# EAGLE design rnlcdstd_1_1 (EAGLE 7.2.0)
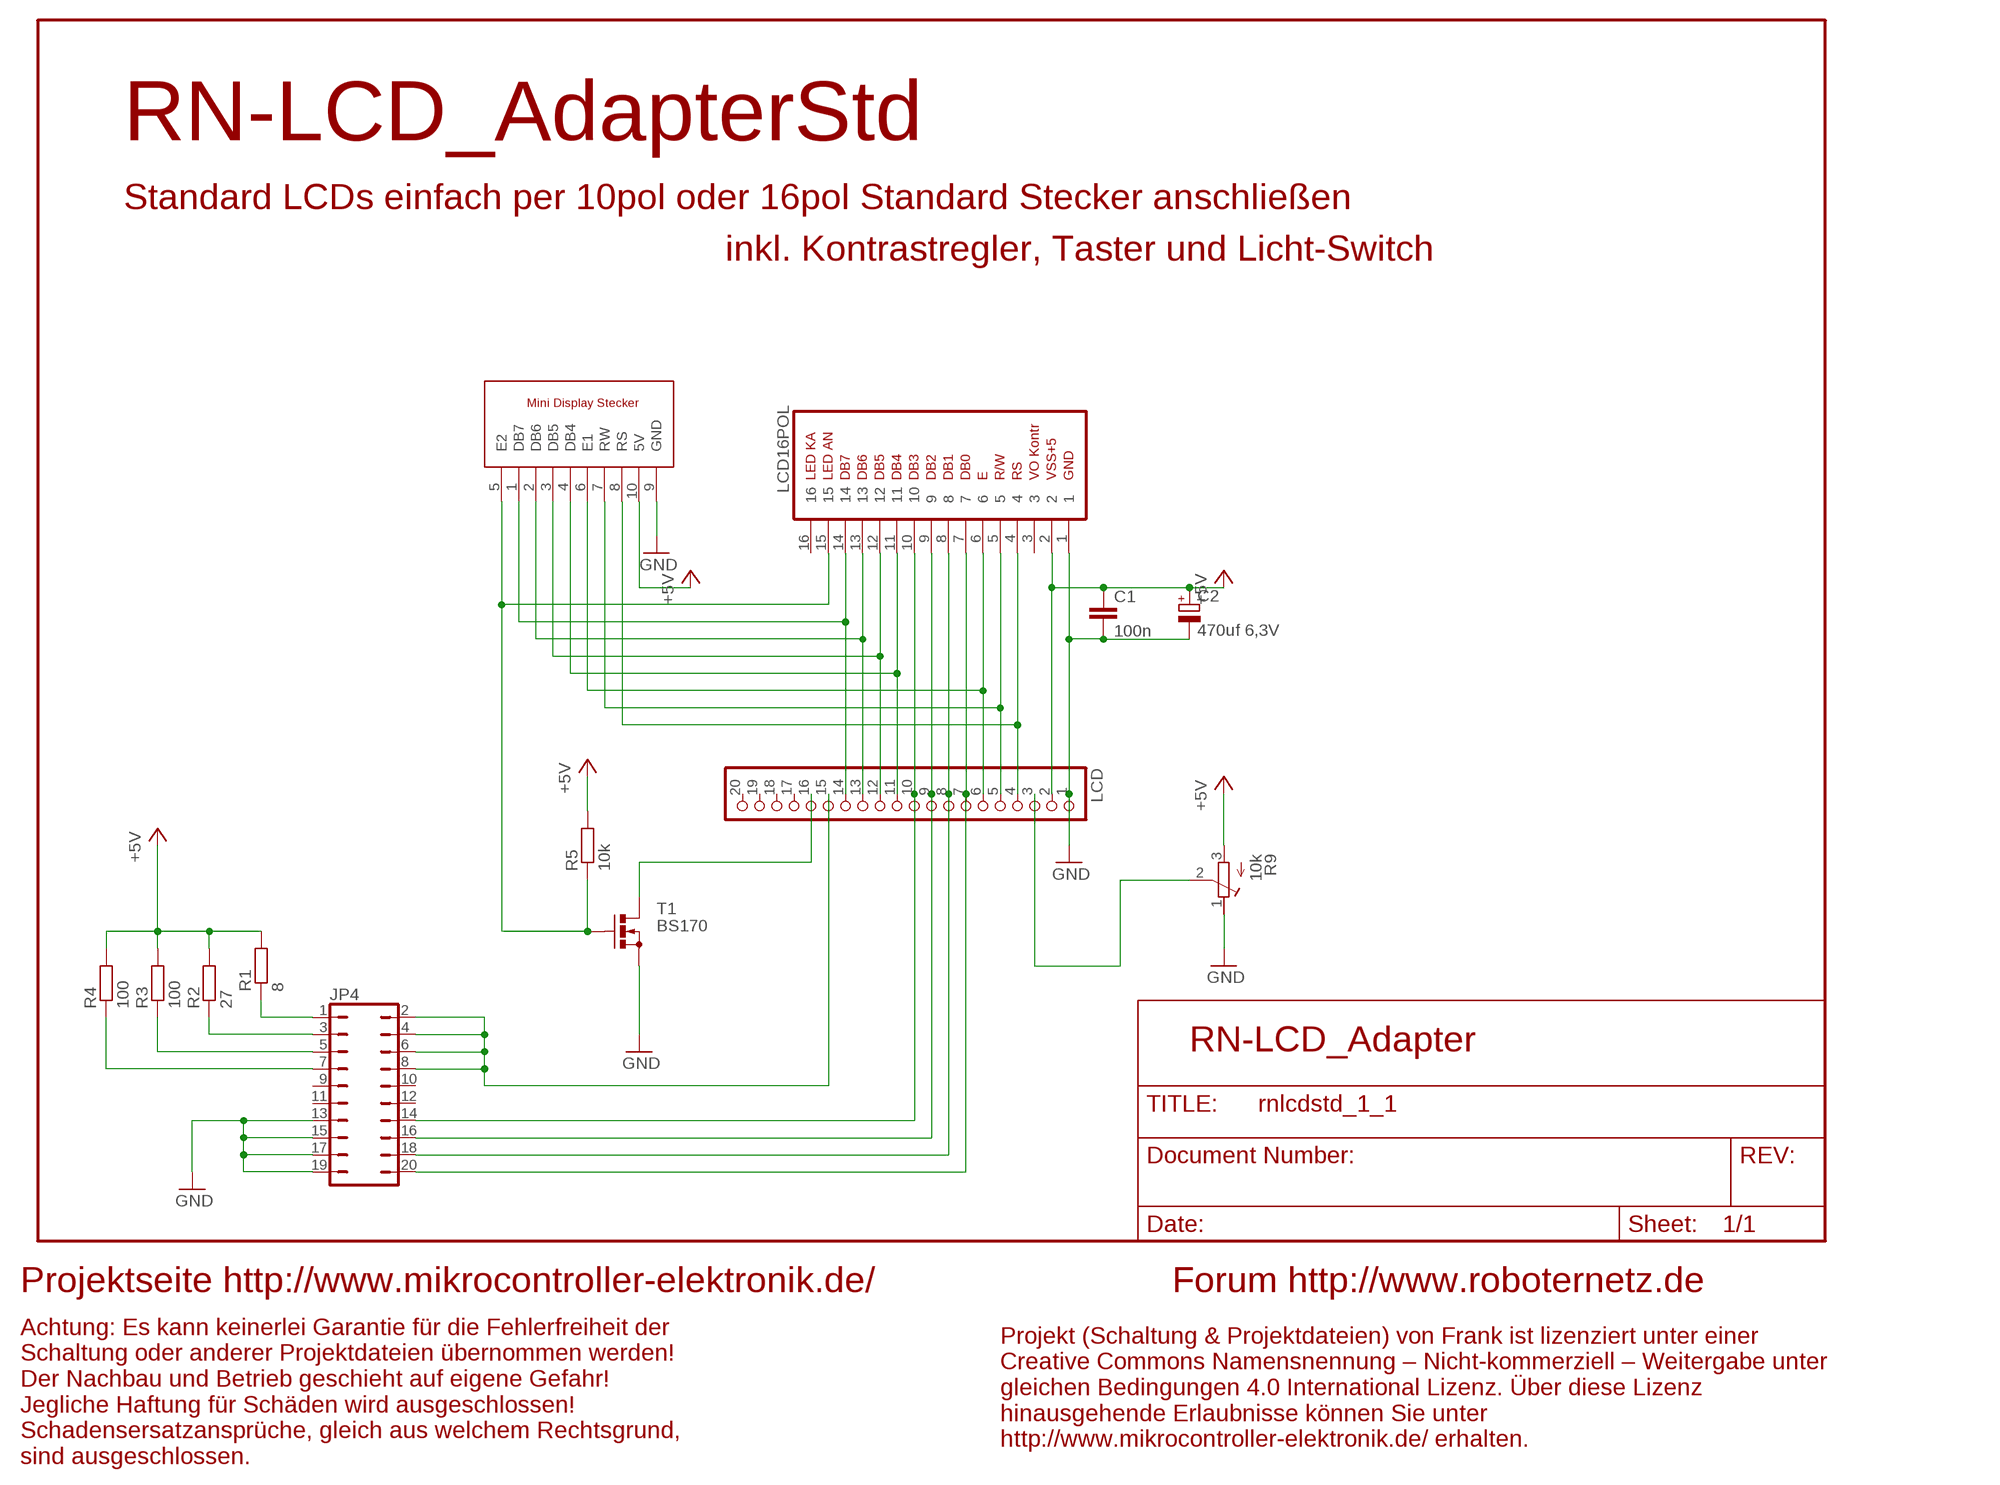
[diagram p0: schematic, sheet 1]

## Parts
C1  100n  C-EU050-024X044  [C050-024X044]
C2  470uf 6,3V  CPOL-EUE3.5-8  [E3,5-8]
JP4  JP10Q  [JP10Q]
LCD  PINHD-1X20  [1X20]
LCD4POL  DISPLAYSTECKER10PNEU  [ML10]
LCD16POL  DISPLAYSTECKER16P  [ML16]
R1  8  R-EU_0309/12  [0309/12]
R2  27  R-EU_0309/12  [0309/12]
R3  100  R-EU_0309/12  [0309/12]
R4  100  R-EU_0309/12  [0309/12]
R5  10k  R-EU_0207/10  [0207/10]
R9  10k  R-TRIMM43P  [RTRIM43P]
T1  BS170  [SOT54E]

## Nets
+5V [power]: C1.1 C2.+ LCD4POL.10(5V) LCD16POL.2 LCD.2 R1.2 R2.2 R3.2 R4.2 R5.2 R9.3(E)
GND [power]: C1.2 C2.- JP4.13 JP4.15 JP4.17 JP4.19 LCD4POL.9(GND) LCD16POL.1 LCD.1 R9.1(A) T1.S
N$1: LCD4POL.1(DB7) LCD16POL.14 LCD.14
N$2 [power]: LCD.16 T1.D
N$3: JP4.2 JP4.4 JP4.6 JP4.8 LCD.15
N$4: JP4.1 R1.1
N$5: LCD4POL.6(E1) LCD16POL.6 LCD.6
N$6: LCD4POL.8(RS) LCD16POL.4 LCD.4
N$7: LCD4POL.7(RW) LCD16POL.5 LCD.5
N$8: LCD.3 R9.2(S)
N$10: JP4.3 R2.1
N$11: JP4.5 R3.1
N$12: JP4.7 R4.1
N$13: LCD4POL.5(E2) LCD16POL.15 R5.1 T1.G
N$14: LCD4POL.2(DB6) LCD16POL.13 LCD.13
N$15: LCD4POL.3(DB5) LCD16POL.12 LCD.12
N$16: LCD4POL.4(DB4) LCD16POL.11 LCD.11
N$17: JP4.20 LCD16POL.7 LCD.7
N$18: JP4.18 LCD16POL.8 LCD.8
N$23: JP4.16 LCD16POL.9 LCD.9
N$24: JP4.14 LCD16POL.10 LCD.10
Unconnected: JP4.9 JP4.10 JP4.11 JP4.12 LCD16POL.3 LCD16POL.16 LCD.17 LCD.18 LCD.19 LCD.20

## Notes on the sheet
- RN-LCD_AdapterStd
- Standard LCDs einfach per 10pol oder 16pol Standard Stecker anschließen
- inkl. Kontrastregler, Taster und Licht-Switch
- RN-LCD_Adapter
- Projektseite http://www.mikrocontroller-elektronik.de/ | Forum http://www.roboternetz.de
- Projekt (Schaltung & Projektdateien) von Frank ist lizenziert unter einer
  Creative Commons Namensnennung – Nicht-kommerziell – Weitergabe unter
  gleichen Bedingungen 4.0 International Lizenz. Über diese Lizenz
  hinausgehende Erlaubnisse können Sie unter
  http://www.mikrocontroller-elektronik.de/ erhalten.
- Achtung: Es kann keinerlei Garantie für die Fehlerfreiheit der
  Schaltung oder anderer Projektdateien übernommen werden!
  Der Nachbau und Betrieb geschieht auf eigene Gefahr! 
  Jegliche Haftung für Schäden wird ausgeschlossen!
  Schadensersatzansprüche, gleich aus welchem Rechtsgrund,
  sind ausgeschlossen.

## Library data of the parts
C1 = rcl:C-EU: CAPACITOR, European symbol
C2 = rcl:CPOL-EU: POLARIZED CAPACITOR, European symbol
JP4 = jumper:JP10Q: JUMPER
LCD = pinhead:PINHD-1X20: PIN HEADER
LCD4POL = RoboterNetz:DISPLAYSTECKER10PNEU
LCD16POL = RoboterNetz:DISPLAYSTECKER16P: HARTING
R1-R5 = rcl:R-EU_: RESISTOR, European symbol
R9 = rcl:R-TRIMM: Trimm resistor
T1 = transistor-small-signal:BS170: N-CHANNEL MOS FET

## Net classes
1 power: width 0.457 mm
2 Power2A: width 0.508 mm
3 Power3A: width 1.016 mm

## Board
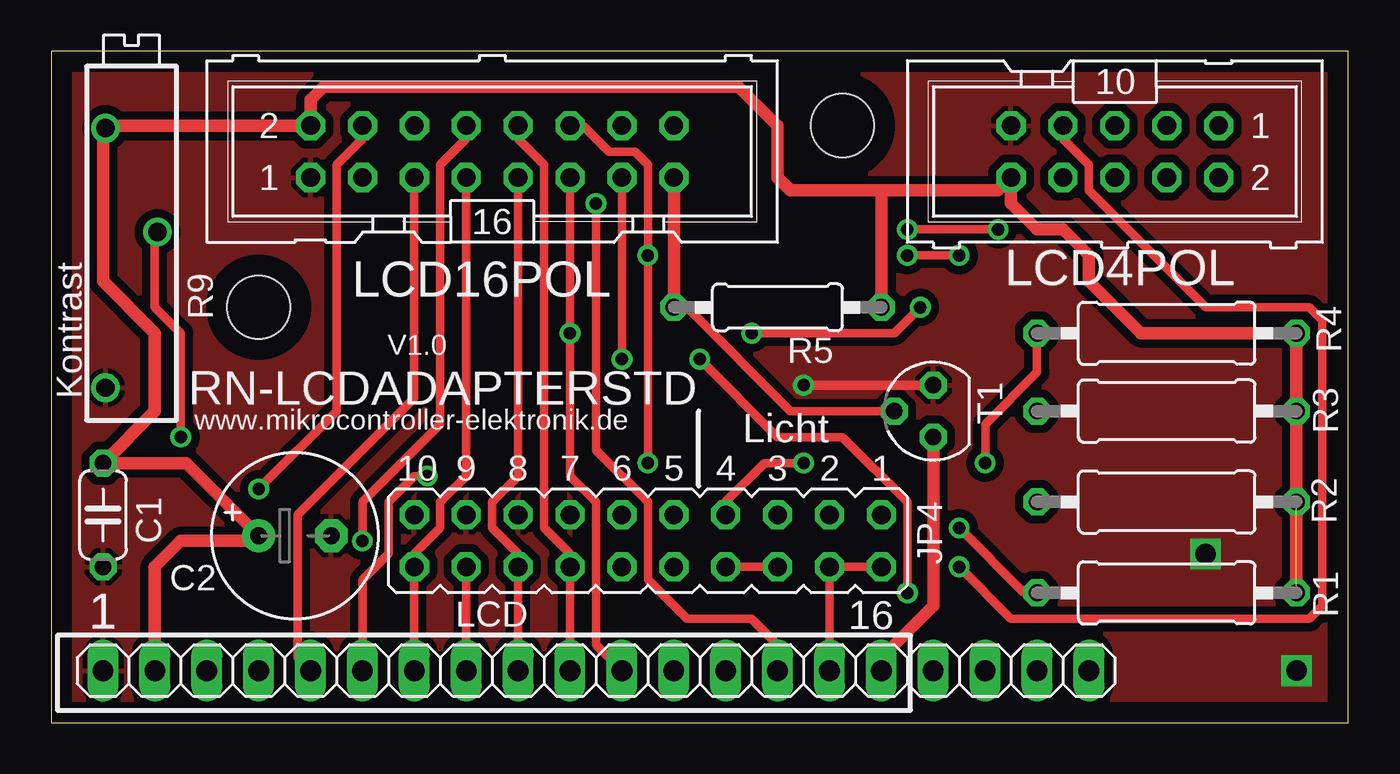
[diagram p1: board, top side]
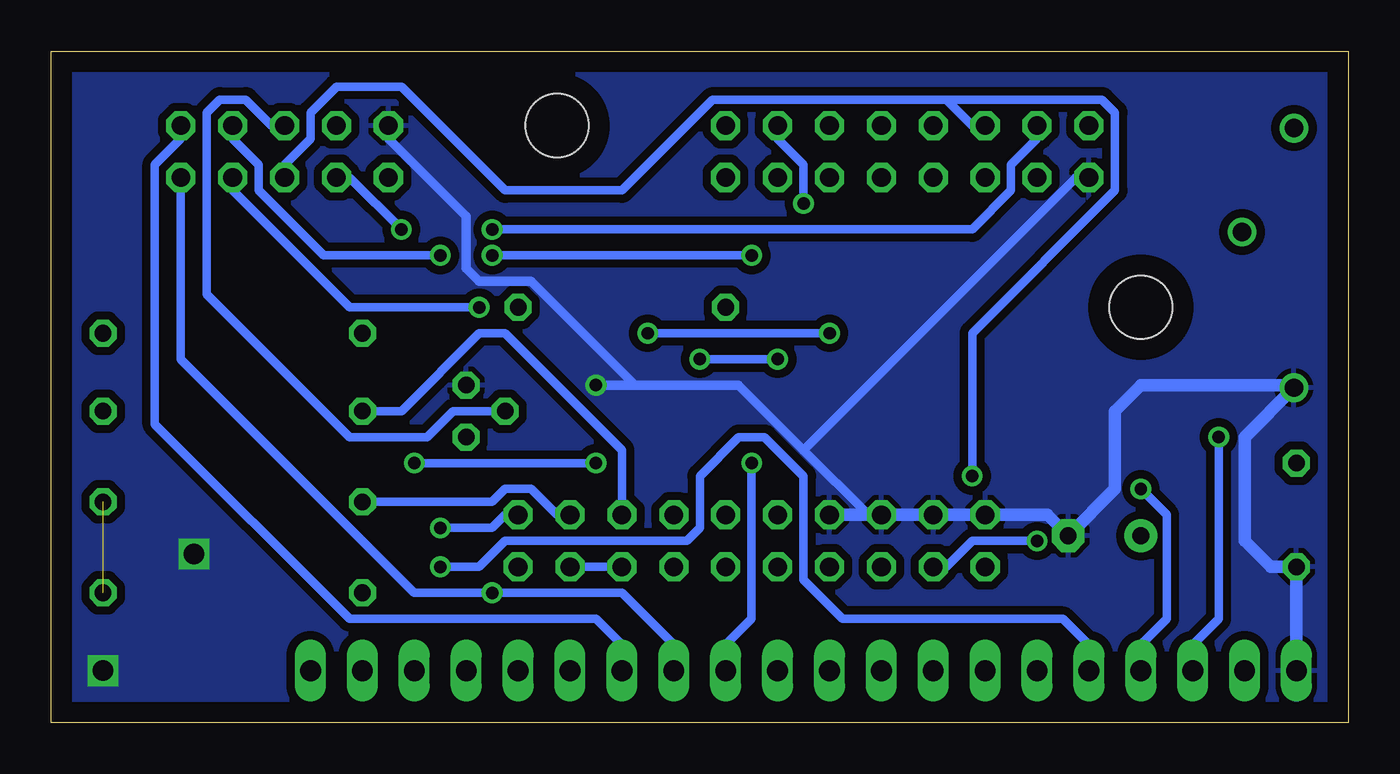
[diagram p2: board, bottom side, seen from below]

Size 63.5 x 32.85 mm. Coordinates in mm from the lower left corner, seen from the top.
Outline: 0,0 63.5,0 63.48,32.85 0.01,32.85 0,0
Copper layers (1*16): Top 0.035mm / dielectric 1.5mm / Bottom 0.035mm
Design rules "default": minimum track width 16mil, minimum drill 24mil, track to track 10mil, track to pad 10mil, pad to pad 10mil, via to via 8mil, smd to smd 8mil, copper to edge 40mil, drill to drill 8mil, minimum pad ring 10mil, minimum via ring 8mil, stop-mask expansion 4mil, vias tented up to drill 0mil, thermal gap 10mil
Holes 3.1 mm at 10.16,20.32 38.73,29.21

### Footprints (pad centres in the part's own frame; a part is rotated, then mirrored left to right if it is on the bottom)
C050-024X044 = drill 0.813 octagon: 1 -2.54,0; 2 2.54,0
E3,5-8 = drill 0.813 pad 1.6: + -1.778,0 | drill 0.813 pad 1.6 octagon: - 1.778,0
JP10Q = drill 0.914 octagon: 1 -11.43,-1.27; 2 -11.43,1.27; 3 -8.89,-1.27; 4 -8.89,1.27; 5 -6.35,-1.27; 6 -6.35,1.27; 7 -3.81,-1.27; 8 -3.81,1.27; 9 -1.27,-1.27; 10 -1.27,1.27; 11 1.27,-1.27; 12 1.27,1.27; 13 3.81,-1.27; 14 3.81,1.27; 15 6.35,-1.27; 16 6.35,1.27; 17 8.89,-1.27; 18 8.89,1.27; 19 11.43,-1.27; 20 11.43,1.27
1X20 = drill 1.016 long: 1 -24.13,0; 2 -21.59,0; 3 -19.05,0; 4 -16.51,0; 5 -13.97,0; 6 -11.43,0; 7 -8.89,0; 8 -6.35,0; 9 -3.81,0; 10 -1.27,0; 11 1.27,0; 12 3.81,0; 13 6.35,0; 14 8.89,0; 15 11.43,0; 16 13.97,0; 17 16.51,0; 18 19.05,0; 19 21.59,0; 20 24.13,0
ML10 = drill 0.914 octagon: 1 -5.08,-1.27; 2 -5.08,1.27; 3 -2.54,-1.27; 4 -2.54,1.27; 5 0,-1.27; 6 0,1.27; 7 2.54,-1.27; 8 2.54,1.27; 9 5.08,-1.27; 10 5.08,1.27
ML16 = drill 0.914 octagon: 1 -8.89,-1.27; 2 -8.89,1.27; 3 -6.35,-1.27; 4 -6.35,1.27; 5 -3.81,-1.27; 6 -3.81,1.27; 7 -1.27,-1.27; 8 -1.27,1.27; 9 1.27,-1.27; 10 1.27,1.27; 11 3.81,-1.27; 12 3.81,1.27; 13 6.35,-1.27; 14 6.35,1.27; 15 8.89,-1.27; 16 8.89,1.27
0309/12 = drill 0.813 octagon: 1 -6.35,0; 2 6.35,0
0207/10 = drill 0.813 octagon: 1 -5.08,0; 2 5.08,0
RTRIM43P = drill 0.9: 1 -7.62,1.27; 2 0,-1.27; 3 5.08,1.27
SOT54E = drill 0.813 octagon: D -1.27,0; G 0,1.905; S 1.27,0

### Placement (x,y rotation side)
C1  2.54,10.16 270 top
C2  11.94,9.14 0 top
JP4  29.21,8.89 180 top
LCD  26.67,2.54 0 top
LCD4POL  52.07,27.94 180 top
LCD16POL  21.59,27.94 0 top
R1  54.61,6.35 0 top
R2  54.61,10.79 0 top
R3  54.61,15.24 0 top
R4  54.61,19.05 0 top
R5  35.56,20.32 0 top
R9  3.94,24 90 top
T1  43.18,15.24 90 top

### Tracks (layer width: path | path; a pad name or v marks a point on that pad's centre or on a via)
+5V  (1 unrouted)
  Top 0.61: LCD.2 5.08,7.62 6.35,8.89 10.16,8.89 C2.+ 6.6,12.7 C1.1 5.08,15.24 5.08,19.05 2.54,21.59 2.54,29.21 R9.3 2.79,29.21 LCD16POL.2 12.7,30.48 13.34,31.11 33.66,31.11 35.56,29.21 35.56,26.67 36.2,26.04 40.64,26.04 | R1.2 R3.2 R4.2 53.34,19.05 50.8,21.59 50.8,22.86 49.53,24.13 48.26,24.13 46.99,25.4 LCD4POL.10 46.35,26.04 40.64,26.04 | 40.64,26.04 R5.2
GND  (via drill 0.61, 1)
  Top 0.457: v36.83,16.51 T1.S
  Bottom 0.457: 34.92,16.51 29.84,16.51 26.67,13.34 | 34.92,16.51 v36.83,16.51 | 23.5,10.16 26.67,13.34 | 26.67,13.34 13.34,26.67 LCD16POL.1 | 34.92,16.51 40.01,21.59 42.55,21.59 43.18,22.23 43.18,24.77 46.99,28.57 LCD4POL.9
  Bottom 0.61: LCD.1 C1.2 3.81,7.62 5.08,8.89 5.08,13.97 R9.1 2.54,16.51 10.16,16.51 11.43,15.24 11.43,11.43 C2.- 14.73,10.16 JP4.19 JP4.17 JP4.15 23.5,10.16 JP4.13
  other vias: 56.52,8.26 60.96,2.54
  pour Bottom (isolate 0.406): 0,0 0,32.38 63.5,32.38 63.5,0
  pour Top (isolate 0.406): 0,0 0,32.38 63.5,32.38 63.5,0
N$1  (via drill 0.61)
  Top 0.406: v26.67,25.4 26.67,13.34 29.21,10.79 29.21,6.99 31.11,5.08 34.29,5.08 35.56,3.81 LCD.14
  Bottom 0.406: v26.67,25.4 26.67,27.3 27.94,28.57 LCD16POL.14 | LCD4POL.1 57.15,28.57 58.42,27.3 58.42,14.61 48.9,5.08 36.83,5.08 35.56,3.81 LCD.14
N$2
  Top 0.61: LCD.16 40.64,3.17 43.18,5.71 T1.D
N$3
  Top 0.406: JP4.8 JP4.6 | JP4.2 JP4.4 LCD.15
  Bottom 0.406: JP4.6 JP4.4
N$4  (via drill 0.61)
  Top 0.406: v44.45,9.53 47.62,6.35 R1.1
  Bottom 0.406: v44.45,9.53 41.91,9.53 41.27,10.16 JP4.1
N$5  (via drill 0.61)
  Top 0.406: v18.41,12.06 17.78,12.06 16.51,10.79 16.51,8.26 15.24,6.99 LCD.6
  Bottom 0.406: 19.68,30.48 31.11,30.48 35.56,26.04 41.27,26.04 46.35,31.11 49.53,31.11 50.8,29.84 50.8,28.57 52.07,27.3 LCD4POL.6 | 19.68,30.48 18.41,29.21 LCD16POL.6 | v18.41,12.06 18.41,19.05 11.43,26.04 11.43,29.84 12.06,30.48 19.68,30.48
N$6  (via drill 0.61)
  Top 0.406: v10.16,11.43 13.97,15.24 13.97,27.3 15.24,28.57 LCD16POL.4 | v41.91,24.13 v46.35,24.13
  Bottom 0.406: v10.16,11.43 8.89,10.16 8.89,5.08 10.16,3.81 LCD.4 | v46.35,24.13 48.9,26.67 LCD4POL.8 | v41.91,24.13 18.41,24.13 16.51,26.04 16.51,27.3 15.24,28.57 LCD16POL.4
N$7  (via drill 0.61)
  Top 0.406: LCD16POL.5 17.78,15.88 12.06,10.16 12.06,3.17 LCD.5 | v44.45,7.62 46.99,5.08 61.59,5.08 62.23,5.71 62.23,19.68 61.59,20.32 56.52,20.32 50.8,26.04 50.8,27.3 49.53,28.57 LCD4POL.7
  Bottom 0.406: v44.45,7.62 42.55,7.62 41.27,8.89 32.38,8.89 31.75,9.53 31.75,12.06 29.84,13.97 28.57,13.97 26.67,12.06 26.67,6.99 24.77,5.08 13.97,5.08 12.7,3.81 LCD.5
N$8  (via drill 0.61)
  Top 0.406: v6.35,13.97 6.35,19.05 5.08,20.32 5.08,23.5 R9.2
  Bottom 0.406: v6.35,13.97 6.35,5.08 7.62,3.81 LCD.3
N$10
  Bottom 0.406: R2.1 41.91,10.79 41.27,11.43 40.01,11.43 38.73,10.16 JP4.3
N$11
  Bottom 0.406: R3.1 46.35,15.24 42.55,19.05 41.27,19.05 35.56,13.34 JP4.5
N$12  (via drill 0.61)
  Top 0.406: v45.72,12.7 45.72,14.61 48.26,17.14 R4.1 | v36.83,12.7 34.92,12.7 33.02,10.79 JP4.7
  Bottom 0.406: v36.83,12.7 v45.72,12.7
N$13
  Top 0.406: T1.G 36.2,15.24 31.11,20.32 R5.1
  Top 0.61: R5.1 LCD16POL.15
  Bottom 0.406: LCD4POL.5 52.7,29.21 53.98,30.48 55.24,30.48 55.88,29.84 55.88,20.95 48.9,13.97 45.09,13.97 43.81,15.24 T1.G
N$14  (via drill 0.61)
  Top 0.406: v31.75,17.78 35.56,13.97 38.73,13.97 41.91,10.79 v41.91,6.35 | v27.94,17.78 LCD16POL.13
  Bottom 0.406: v31.75,17.78 v27.94,17.78 | LCD.13 33.02,3.81 35.56,6.35 v41.91,6.35 45.72,6.35 57.15,17.78 LCD4POL.2
N$15  (via drill 0.61)
  Top 0.406: v29.21,12.7 v29.21,22.86 29.21,27.3 28.57,27.94 27.3,27.94 26.04,29.21 LCD16POL.12 | v41.91,22.86 v44.45,22.86
  Bottom 0.406: v29.21,12.7 29.21,5.08 30.48,3.81 LCD.12 | v44.45,22.86 50.16,22.86 53.34,26.04 53.34,27.3 54.61,28.57 LCD4POL.3 | v29.21,22.86 v41.91,22.86
N$16  (via drill 0.61)
  Top 0.406: LCD16POL.11 v25.4,19.05 25.4,12.06 26.67,10.79 26.67,3.81 LCD.11 | v42.55,20.32 41.27,19.05 v34.29,19.05
  Bottom 0.406: v42.55,20.32 48.9,20.32 54.61,26.04 LCD4POL.4 | v25.4,19.05 v34.29,19.05
N$17
  Top 0.406: LCD.7 JP4.20 17.78,8.26 19.05,9.53 19.05,10.79 20.32,12.06 LCD16POL.7
N$18  (via drill 0.61)
  Top 0.406: LCD.8 JP4.18 | v15.24,8.89 15.24,10.79 19.05,14.61 19.05,27.3 20.32,28.57 LCD16POL.8
  Bottom 0.406: v15.24,8.89 18.41,8.89 19.68,7.62 JP4.18
N$23
  Top 0.406: LCD.9 JP4.16 22.86,8.26 21.59,9.53 21.59,10.79 22.86,12.06 LCD16POL.9
N$24
  Top 0.406: LCD.10 JP4.14 25.4,8.26 24.13,9.53 24.13,27.3 22.86,28.57 LCD16POL.10

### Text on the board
tPlace: V1.0 | Kontrast | RN-LCDADAPTERSTD | www.mikrocontroller-elektronik.de | Licht | 1 | 16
